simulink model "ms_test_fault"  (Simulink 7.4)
settings: Solver=ode23t  StartTime=0.0  StopTime=15  RelTol=1e-5
undefined symbols (not defined in the file or in its folder): D1, Delta, dfilt, DiscIntNeverNeededParam
libraries: powerlib x47, simulink x12, powerlib_extras x8, dsparch4 x3
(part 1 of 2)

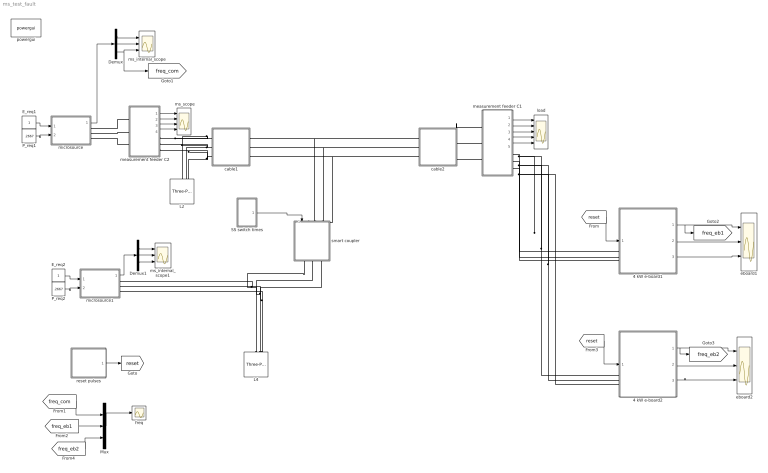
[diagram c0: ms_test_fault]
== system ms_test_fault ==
  " ms_scope" : Scope  NumInputPorts=4
  4 kW e-board1 : Subsystem  mask{tf=100, p=1}
      mask prompts: tf "fault_time"; p "load priority"
  4 kW e-board2 : Subsystem  mask{tf=100, p=2}
      mask prompts: tf "fault time"; p "priority level"
  Demux : Demux  Outputs=3
  Demux1 : Demux  Outputs=3
  E_req1 : Constant  OutDataType=fixdt(1, 16)  OutScaling=2^0
  E_req2 : Constant  OutDataType=fixdt(1, 16)  OutScaling=2^0
  L2 : powerlib/Elements/Three-Phase Series RLC Load  DialogController=POWERSYS.PowerSysDialog  PhysicalDomain=powersysdomain  SubClassName=unknown  LeftPortType=p1  RightPortType=p1  LConnTagsString=A|B|C  Configuration=Y (grounded)  NominalVoltage=208  NominalFrequency=60  ActivePower=4000  InductivePower=0  CapacitivePower=0  Measurements=None
  L4 : powerlib/Elements/Three-Phase Series RLC Load  DialogController=POWERSYS.PowerSysDialog  PhysicalDomain=powersysdomain  SubClassName=unknown  LeftPortType=p1  RightPortType=p1  LConnTagsString=A|B|C  Configuration=Y (grounded)  NominalVoltage=208  NominalFrequency=60  ActivePower=4000  InductivePower=0  CapacitivePower=0  Measurements=None
  Mux : Mux  Inputs=3
  P_req1 : Constant  Value=.2667  OutDataType=fixdt(1, 16)  OutScaling=2^0
  P_req2 : Constant  Value=.2667  OutDataType=fixdt(1, 16)  OutScaling=2^0
  SS switch times : Subsystem  mask{tdisconnect=3, dt=4}
      mask prompts: tdisconnect "disconnect time"; dt "disconnection interval"
  cable1 : Subsystem  mask{R=.002657, L=.000641, C=2020}
  cable2 : Subsystem  mask{R=0.0168, L=0.00407, C=336}
  eboard1 : Scope  NumInputPorts=3
  eboard2 : Scope  NumInputPorts=3
  freq : Scope
  load : Scope  NumInputPorts=5
  measurement feeder C1 : Subsystem
  measurement feeder C2 : Subsystem
  microsource : Subsystem  AncestorBlock=|
      | UWM_blocks/inverter-based
      | DG (simplified)
      | 208V - 15kVA
  microsource1 : Subsystem  AncestorBlock=|
      | UWM_blocks/inverter-based
      | DG (simplified)
      | 208V - 15kVA
  ms_internal_scope : Scope  NumInputPorts=3
  ms_internal_scope1 : Scope  NumInputPorts=3
  powergui : powerlib/powergui  Priority=1  SystemSampleTime=-1  SimulationMode=Discrete  SampleTime=50e-6  frequency=60  SPID=off  DisableSnubberDevices=off  DisableRonSwitches=off  DisableVfSwitches=off  SwTol=0  Interpol=off  frequencyindice=0  echomessages=off  HookPort=off  DisplayEquations=off  FunctionMessages=off  EnableUseOfTLC=off  x0status=blocks  RestoreLinks=warning  Frange=[0:2:500]  Ylog=off  Xlog=on  ShowGrid=off  save=off  variable=ZData  ZoomFFT=on  StartTime=0.0  cycles=1  DisplayStyle=1  fundamental=60  FreqAxis=off  MaxFrequency=1000  frequencyindicesteady=1  RmsSteady=1  display=off  Ts=0  methode=off
  reset pulses : Subsystem  mask{tpulse=[2 100]}
  smart coupler : Subsystem
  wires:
  measurement feeder C2/1(Vabc) -> " ms_scope"/1
  measurement feeder C2/2(Iabc) -> " ms_scope"/2
  measurement feeder C2/3(PQ) -> " ms_scope"/3
  measurement feeder C2/4(RMS (V-I)) -> " ms_scope"/4
  measurement feeder C1/5(w) -> load/5
  measurement feeder C1/4(RMS (V-I)) -> load/4
  measurement feeder C1/3(PQ) -> load/3
  measurement feeder C1/2(Iabc) -> load/2
  measurement feeder C1/1(Vabc) -> load/1
  P_req1/1 -> microsource/2(P_req)
  E_req1/1 -> microsource/1(E_req)
  Demux/2 -> ms_internal_scope/2
  Demux/1 -> ms_internal_scope/1
  Demux/3 -> ms_internal_scope/3, [freq_com]
  microsource/1(m) -> Demux/1
  Mux/1 -> freq/1
  P_req2/1 -> microsource1/2(P_req)
  E_req2/1 -> microsource1/1(E_req)
  microsource1/1(m) -> Demux1/1
  Demux1/1 -> ms_internal_scope1/1
  Demux1/2 -> ms_internal_scope1/2
  Demux1/3 -> ms_internal_scope1/3
  4 kW e-board1/1(w) -> eboard1/1, [freq_eb1]
  reset pulses/1(Out1) -> [reset]
  [reset] -> 4 kW e-board1/1(reset)
  [freq_com] -> Mux/1
  4 kW e-board1/2(Irms) -> eboard1/2
  4 kW e-board1/3(Vrms) -> eboard1/3
  [freq_eb1] -> Mux/2
  [reset] -> 4 kW e-board2/1(reset)
  4 kW e-board2/1(w) -> eboard2/1, [freq_eb2]
  4 kW e-board2/2(Irms) -> eboard2/2
  4 kW e-board2/3(Vrms) -> eboard2/3
  [freq_eb2] -> Mux/3
  SS switch times/1(Out1) -> smart coupler/1(switch)
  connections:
  cable1/RConn1 -- L2/LConn1 -- measurement feeder C2/RConn1
  cable1/RConn2 -- L2/LConn2 -- measurement feeder C2/RConn2
  cable1/RConn3 -- L2/LConn3 -- measurement feeder C2/RConn3
  microsource/RConn1 -- measurement feeder C2/LConn1
  microsource/RConn2 -- measurement feeder C2/LConn2
  microsource/RConn3 -- measurement feeder C2/LConn3
  cable2/LConn1 -- measurement feeder C1/LConn1
  cable2/LConn2 -- measurement feeder C1/LConn2
  cable2/LConn3 -- measurement feeder C1/LConn3
  measurement feeder C1/RConn1 -- 4 kW e-board1/LConn1 -- 4 kW e-board2/LConn1
  measurement feeder C1/RConn2 -- 4 kW e-board1/LConn2 -- 4 kW e-board2/LConn2
  measurement feeder C1/RConn3 -- 4 kW e-board1/LConn3 -- 4 kW e-board2/LConn3
  cable2/RConn2 -- cable1/LConn2 -- smart coupler/LConn2
  cable2/RConn3 -- cable1/LConn3 -- smart coupler/LConn3
  L4/LConn2 -- microsource1/RConn2 -- smart coupler/RConn2
  L4/LConn3 -- microsource1/RConn3 -- smart coupler/RConn3
  cable2/RConn1 -- cable1/LConn1 -- smart coupler/LConn1
  L4/LConn1 -- microsource1/RConn1 -- smart coupler/RConn1

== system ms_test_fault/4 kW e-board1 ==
  reset : Inport
  Current Measurement : powerlib/Measurements/Current Measurement  DialogController=POWERSYS.PowerSysDialog  SystemSampleTime=-1  PhasorSimulation=off  OutputType=Complex  PSBequivalent=0
  Ground : powerlib/Elements/Ground  DialogController=POWERSYS.PowerSysDialog  PhysicalDomain=powersysdomain  SubClassName=unknown  LeftPortType=p1  RightPortType=p1  LConnTagsString=a
  L1 : powerlib/Elements/Three-Phase Series RLC Load  DialogController=POWERSYS.PowerSysDialog  PhysicalDomain=powersysdomain  SubClassName=unknown  LeftPortType=p1  RightPortType=p1  LConnTagsString=A|B|C  Configuration=Y (grounded)  NominalVoltage=208  NominalFrequency=60  ActivePower=4000  InductivePower=0  CapacitivePower=0  Measurements=None
  Three-Phase Breaker2 : powerlib/Elements/Three-Phase Breaker  DialogController=POWERSYS.PowerSysDialog  SystemSampleTime=-1  InitialState=closed  SwitchA=on  SwitchB=on  SwitchC=on  SwitchTimes=[50]  External=on  BreakerResistance=0.001  SnubberResistance=1e6  SnubberCapacitance=inf  Measurements=None
  Three-Phase Fault : powerlib/Elements/Three-Phase Fault  DialogController=POWERSYS.PowerSysDialog  SystemSampleTime=-1  FaultA=on  FaultB=on  FaultC=on  FaultResistance=0.001  GroundFault=on  GroundResistance=0.001  External=off  SwitchStatus=[1 0]  SwitchTimes=[tf tf+3/60]  InitialStates=[0 0 1]  SnubberResistance=1e6  SnubberCapacitance=inf  Measurements=None
  Voltage  Measurement : powerlib/Measurements/Voltage Measurement  DialogController=POWERSYS.PowerSysDialog  SystemSampleTime=-1  PhasorSimulation=off  OutputType=Complex  PSBequivalent=0
  trip : Subsystem  mask{p=p}
      mask prompts: p "priority level"
  A : PMIOPort  Port=1  Side=Left
  B : PMIOPort  Port=2  Side=Left
  C : PMIOPort  Port=3  Side=Left
  w : Outport  OutDataType=fixdt(1, 16)  OutScaling=2^0
  Irms : Outport  Port=2  OutDataType=fixdt(1, 16)  OutScaling=2^0
  Vrms : Outport  Port=3  OutDataType=fixdt(1, 16)  OutScaling=2^0
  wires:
  trip/1(w) -> w/1
  Current Measurement/1 -> trip/3(I)
  Voltage  Measurement/1 -> trip/2(V)
  reset/1 -> trip/1(Reset)
  trip/2(trip) -> Three-Phase Breaker2/1
  trip/3(Irms) -> Irms/1
  trip/4(Vrms) -> Vrms/1
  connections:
  A/RConn1 -- Current Measurement/LConn1 -- Voltage  Measurement/LConn1
  Voltage  Measurement/LConn2 -- Ground/LConn1
  B/RConn1 -- Three-Phase Breaker2/LConn2
  Current Measurement/RConn1 -- Three-Phase Breaker2/LConn1
  C/RConn1 -- Three-Phase Breaker2/LConn3
  Three-Phase Breaker2/RConn1 -- Three-Phase Fault/LConn1 -- L1/LConn1
  Three-Phase Breaker2/RConn2 -- Three-Phase Fault/LConn2 -- L1/LConn2
  Three-Phase Breaker2/RConn3 -- Three-Phase Fault/LConn3 -- L1/LConn3

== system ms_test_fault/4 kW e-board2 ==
  reset : Inport
  Current Measurement : powerlib/Measurements/Current Measurement  DialogController=POWERSYS.PowerSysDialog  SystemSampleTime=-1  PhasorSimulation=off  OutputType=Complex  PSBequivalent=0
  Ground : powerlib/Elements/Ground  DialogController=POWERSYS.PowerSysDialog  PhysicalDomain=powersysdomain  SubClassName=unknown  LeftPortType=p1  RightPortType=p1  LConnTagsString=a
  L1 : powerlib/Elements/Three-Phase Series RLC Load  DialogController=POWERSYS.PowerSysDialog  PhysicalDomain=powersysdomain  SubClassName=unknown  LeftPortType=p1  RightPortType=p1  LConnTagsString=A|B|C  Configuration=Y (grounded)  NominalVoltage=208  NominalFrequency=60  ActivePower=4000  InductivePower=0  CapacitivePower=0  Measurements=None
  Three-Phase Breaker2 : powerlib/Elements/Three-Phase Breaker  DialogController=POWERSYS.PowerSysDialog  SystemSampleTime=-1  InitialState=closed  SwitchA=on  SwitchB=on  SwitchC=on  SwitchTimes=[50]  External=on  BreakerResistance=0.001  SnubberResistance=1e6  SnubberCapacitance=inf  Measurements=None
  Three-Phase Fault : powerlib/Elements/Three-Phase Fault  DialogController=POWERSYS.PowerSysDialog  SystemSampleTime=-1  FaultA=on  FaultB=on  FaultC=on  FaultResistance=0.001  GroundFault=on  GroundResistance=0.001  External=off  SwitchStatus=[1 0]  SwitchTimes=[tf tf+3/60]  InitialStates=[0 0 1]  SnubberResistance=1e6  SnubberCapacitance=inf  Measurements=None
  Voltage  Measurement : powerlib/Measurements/Voltage Measurement  DialogController=POWERSYS.PowerSysDialog  SystemSampleTime=-1  PhasorSimulation=off  OutputType=Complex  PSBequivalent=0
  trip : Subsystem  mask{p=p}
      mask prompts: p "priority level"
  A : PMIOPort  Port=1  Side=Left
  B : PMIOPort  Port=2  Side=Left
  C : PMIOPort  Port=3  Side=Left
  w : Outport  OutDataType=fixdt(1, 16)  OutScaling=2^0
  Irms : Outport  Port=2  OutDataType=fixdt(1, 16)  OutScaling=2^0
  Vrms : Outport  Port=3  OutDataType=fixdt(1, 16)  OutScaling=2^0
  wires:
  trip/1(w) -> w/1
  Current Measurement/1 -> trip/3(I)
  Voltage  Measurement/1 -> trip/2(V)
  reset/1 -> trip/1(Reset)
  trip/2(trip) -> Three-Phase Breaker2/1
  trip/3(Irms) -> Irms/1
  trip/4(Vrms) -> Vrms/1
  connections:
  A/RConn1 -- Current Measurement/LConn1 -- Voltage  Measurement/LConn1
  Voltage  Measurement/LConn2 -- Ground/LConn1
  B/RConn1 -- Three-Phase Breaker2/LConn2
  Current Measurement/RConn1 -- Three-Phase Breaker2/LConn1
  C/RConn1 -- Three-Phase Breaker2/LConn3
  Three-Phase Breaker2/RConn1 -- Three-Phase Fault/LConn1 -- L1/LConn1
  Three-Phase Breaker2/RConn2 -- Three-Phase Fault/LConn2 -- L1/LConn2
  Three-Phase Breaker2/RConn3 -- Three-Phase Fault/LConn3 -- L1/LConn3

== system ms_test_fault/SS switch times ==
  Sum : Sum  Inputs=|++  OutDataType=fixdt(1, 16)  OutScaling=2^0
  disconnect : Step  Time=tdisconnect  Before=1  After=0  SampleTime=0
  reconnect : Step  Time=tdisconnect+dt  SampleTime=0
  Out1 : Outport
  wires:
  reconnect/1 -> Sum/2
  disconnect/1 -> Sum/1
  Sum/1 -> Out1/1

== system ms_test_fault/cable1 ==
  Ground1 : powerlib/Elements/Ground  DialogController=POWERSYS.PowerSysDialog  PhysicalDomain=powersysdomain  SubClassName=unknown  LeftPortType=p1  RightPortType=p1  LConnTagsString=a
  Three-Phase Parallel RLC Branch : powerlib/Elements/Three-Phase Parallel RLC Branch  DialogController=POWERSYS.PowerSysDialog  PhysicalDomain=powersysdomain  SubClassName=unknown  LeftPortType=p1  RightPortType=p1  LConnTagsString=A|B|C  RConnTagsString=A|B|C  BranchType=C  Resistance=1  Inductance=1e-3  Capacitance=1/(C*2*pi*60)  Measurements=None
  Three-Phase Series RLC Branch3 : powerlib/Elements/Three-Phase Series RLC Branch  DialogController=POWERSYS.PowerSysDialog  PhysicalDomain=powersysdomain  SubClassName=unknown  LeftPortType=p1  RightPortType=p1  LConnTagsString=A|B|C  RConnTagsString=A|B|C  BranchType=RL  Resistance=R  Inductance=L/(2*pi*60)  Capacitance=1/(336*2*pi*60)  Measurements=None
  A* : PMIOPort  Tag=PMCPort  Port=1  Side=Right
  B* : PMIOPort  Tag=PMCPort  Port=2  Side=Right
  C* : PMIOPort  Tag=PMCPort  Port=3  Side=Right
  A : PMIOPort  Tag=PMCPort  Port=4  Side=Left
  B : PMIOPort  Tag=PMCPort  Port=5  Side=Left
  C : PMIOPort  Tag=PMCPort  Port=6  Side=Left
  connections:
  Three-Phase Parallel RLC Branch/RConn3 -- Ground1/LConn1 -- Three-Phase Parallel RLC Branch/RConn2 -- Three-Phase Parallel RLC Branch/RConn1
  Three-Phase Parallel RLC Branch/LConn1 -- A*/RConn1 -- Three-Phase Series RLC Branch3/LConn1
  Three-Phase Parallel RLC Branch/LConn2 -- B*/RConn1 -- Three-Phase Series RLC Branch3/LConn2
  Three-Phase Parallel RLC Branch/LConn3 -- C*/RConn1 -- Three-Phase Series RLC Branch3/LConn3
  A/RConn1 -- Three-Phase Series RLC Branch3/RConn1
  B/RConn1 -- Three-Phase Series RLC Branch3/RConn2
  C/RConn1 -- Three-Phase Series RLC Branch3/RConn3

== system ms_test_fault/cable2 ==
  Ground1 : powerlib/Elements/Ground  DialogController=POWERSYS.PowerSysDialog  PhysicalDomain=powersysdomain  SubClassName=unknown  LeftPortType=p1  RightPortType=p1  LConnTagsString=a
  Three-Phase Parallel RLC Branch : powerlib/Elements/Three-Phase Parallel RLC Branch  DialogController=POWERSYS.PowerSysDialog  PhysicalDomain=powersysdomain  SubClassName=unknown  LeftPortType=p1  RightPortType=p1  LConnTagsString=A|B|C  RConnTagsString=A|B|C  BranchType=C  Resistance=1  Inductance=1e-3  Capacitance=1/(C*2*pi*60)  Measurements=None
  Three-Phase Series RLC Branch3 : powerlib/Elements/Three-Phase Series RLC Branch  DialogController=POWERSYS.PowerSysDialog  PhysicalDomain=powersysdomain  SubClassName=unknown  LeftPortType=p1  RightPortType=p1  LConnTagsString=A|B|C  RConnTagsString=A|B|C  BranchType=RL  Resistance=R  Inductance=L/(2*pi*60)  Capacitance=1/(336*2*pi*60)  Measurements=None
  A* : PMIOPort  Tag=PMCPort  Port=1  Side=Right
  B* : PMIOPort  Tag=PMCPort  Port=2  Side=Right
  C* : PMIOPort  Tag=PMCPort  Port=3  Side=Right
  A : PMIOPort  Tag=PMCPort  Port=4  Side=Left
  B : PMIOPort  Tag=PMCPort  Port=5  Side=Left
  C : PMIOPort  Tag=PMCPort  Port=6  Side=Left
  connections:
  Three-Phase Parallel RLC Branch/RConn3 -- Ground1/LConn1 -- Three-Phase Parallel RLC Branch/RConn2 -- Three-Phase Parallel RLC Branch/RConn1
  Three-Phase Parallel RLC Branch/LConn1 -- A*/RConn1 -- Three-Phase Series RLC Branch3/LConn1
  Three-Phase Parallel RLC Branch/LConn2 -- B*/RConn1 -- Three-Phase Series RLC Branch3/LConn2
  Three-Phase Parallel RLC Branch/LConn3 -- C*/RConn1 -- Three-Phase Series RLC Branch3/LConn3
  A/RConn1 -- Three-Phase Series RLC Branch3/RConn1
  B/RConn1 -- Three-Phase Series RLC Branch3/RConn2
  C/RConn1 -- Three-Phase Series RLC Branch3/RConn3

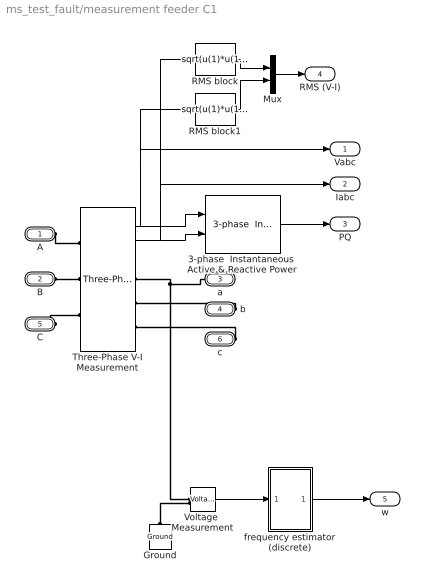
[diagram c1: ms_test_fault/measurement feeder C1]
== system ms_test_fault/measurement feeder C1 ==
  3-phase  Instantaneous  Active & Reactive Power : powerlib_extras/Measurements/3-phase  Instantaneous  Active & Reactive Power  DialogController=POWERSYS.PowerSysDialog  SystemSampleTime=-1
  Ground : powerlib/Elements/Ground  DialogController=POWERSYS.PowerSysDialog  PhysicalDomain=powersysdomain  SubClassName=unknown  LeftPortType=p1  RightPortType=p1  LConnTagsString=a
  Mux : Mux  Inputs=2
  RMS block : Fcn  Expr=sqrt(u(1)*u(1)+u(2)*u(2)+u(3)*u(3))/sqrt(3)
  RMS block1 : Fcn  Expr=sqrt(u(1)*u(1)+u(2)*u(2)+u(3)*u(3))/sqrt(3)
  Three-Phase V-I Measurement : powerlib/Measurements/Three-Phase V-I Measurement  DialogController=POWERSYS.PowerSysDialog  SystemSampleTime=-1  VoltageMeasurement=phase-to-ground  SetLabelV=off  LabelV=Vabc  Vpu=off  CurrentMeasurement=yes  SetLabelI=off  LabelI=Iabc  Ipu=off  Pbase=100e6  Vbase=500e3  OutputType=Complex  PhasorSimulation=off  PSBequivalent=0
  Voltage  Measurement : powerlib/Measurements/Voltage Measurement  DialogController=POWERSYS.PowerSysDialog  SystemSampleTime=-1  PhasorSimulation=off  OutputType=Complex  PSBequivalent=0
  frequency estimator (discrete) : Subsystem  mask{dt=0.010}
      mask prompts: dt "sample time"
  A : PMIOPort  Port=1  Side=Left
  B : PMIOPort  Port=2  Side=Left
  a : PMIOPort  Port=3  Side=Right
  b : PMIOPort  Port=4  Side=Right
  C : PMIOPort  Port=5  Side=Left
  c : PMIOPort  Port=6  Side=Right
  Vabc : Outport  OutDataType=fixdt(1, 16)  OutScaling=2^0
  Iabc : Outport  Port=2  OutDataType=fixdt(1, 16)  OutScaling=2^0
  PQ : Outport  Port=3  OutDataType=fixdt(1, 16)  OutScaling=2^0
  RMS (V-I) : Outport  Port=4  OutDataType=fixdt(1, 16)  OutScaling=2^0
  w : Outport  Port=5  OutDataType=fixdt(1, 16)  OutScaling=2^0
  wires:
  Three-Phase V-I Measurement/1 -> Vabc/1, RMS block1/1, 3-phase  Instantaneous  Active & Reactive Power/1
  Three-Phase V-I Measurement/2 -> Iabc/1, RMS block/1, 3-phase  Instantaneous  Active & Reactive Power/2
  Mux/1 -> RMS (V-I)/1
  RMS block/1 -> Mux/1
  RMS block1/1 -> Mux/2
  3-phase  Instantaneous  Active & Reactive Power/1 -> PQ/1
  Voltage  Measurement/1 -> frequency estimator (discrete)/1(In1)
  frequency estimator (discrete)/1(w) -> w/1
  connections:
  c/RConn1 -- Three-Phase V-I Measurement/RConn3
  C/RConn1 -- Three-Phase V-I Measurement/LConn3
  b/RConn1 -- Three-Phase V-I Measurement/RConn2
  Voltage  Measurement/LConn1 -- a/RConn1 -- Three-Phase V-I Measurement/RConn1
  B/RConn1 -- Three-Phase V-I Measurement/LConn2
  A/RConn1 -- Three-Phase V-I Measurement/LConn1
  Ground/LConn1 -- Voltage  Measurement/LConn2

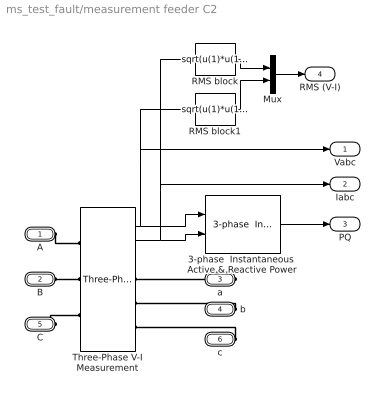
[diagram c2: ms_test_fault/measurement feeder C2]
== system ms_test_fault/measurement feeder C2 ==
  3-phase  Instantaneous  Active & Reactive Power : powerlib_extras/Measurements/3-phase  Instantaneous  Active & Reactive Power  DialogController=POWERSYS.PowerSysDialog  SystemSampleTime=-1
  Mux : Mux  Inputs=2
  RMS block : Fcn  Expr=sqrt(u(1)*u(1)+u(2)*u(2)+u(3)*u(3))/sqrt(3)
  RMS block1 : Fcn  Expr=sqrt(u(1)*u(1)+u(2)*u(2)+u(3)*u(3))/sqrt(3)
  Three-Phase V-I Measurement : powerlib/Measurements/Three-Phase V-I Measurement  DialogController=POWERSYS.PowerSysDialog  SystemSampleTime=-1  VoltageMeasurement=phase-to-ground  SetLabelV=off  LabelV=Vabc  Vpu=off  CurrentMeasurement=yes  SetLabelI=off  LabelI=Iabc  Ipu=off  Pbase=100e6  Vbase=500e3  OutputType=Complex  PhasorSimulation=off  PSBequivalent=0
  A : PMIOPort  Port=1  Side=Left
  B : PMIOPort  Port=2  Side=Left
  a : PMIOPort  Port=3  Side=Right
  b : PMIOPort  Port=4  Side=Right
  C : PMIOPort  Port=5  Side=Left
  c : PMIOPort  Port=6  Side=Right
  Vabc : Outport  OutDataType=fixdt(1, 16)  OutScaling=2^0
  Iabc : Outport  Port=2  OutDataType=fixdt(1, 16)  OutScaling=2^0
  PQ : Outport  Port=3  OutDataType=fixdt(1, 16)  OutScaling=2^0
  RMS (V-I) : Outport  Port=4  OutDataType=fixdt(1, 16)  OutScaling=2^0
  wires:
  Three-Phase V-I Measurement/1 -> Vabc/1, RMS block1/1, 3-phase  Instantaneous  Active & Reactive Power/1
  Three-Phase V-I Measurement/2 -> Iabc/1, RMS block/1, 3-phase  Instantaneous  Active & Reactive Power/2
  Mux/1 -> RMS (V-I)/1
  RMS block/1 -> Mux/1
  RMS block1/1 -> Mux/2
  3-phase  Instantaneous  Active & Reactive Power/1 -> PQ/1
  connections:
  c/RConn1 -- Three-Phase V-I Measurement/RConn3
  C/RConn1 -- Three-Phase V-I Measurement/LConn3
  b/RConn1 -- Three-Phase V-I Measurement/RConn2
  a/RConn1 -- Three-Phase V-I Measurement/RConn1
  B/RConn1 -- Three-Phase V-I Measurement/LConn2
  A/RConn1 -- Three-Phase V-I Measurement/LConn1

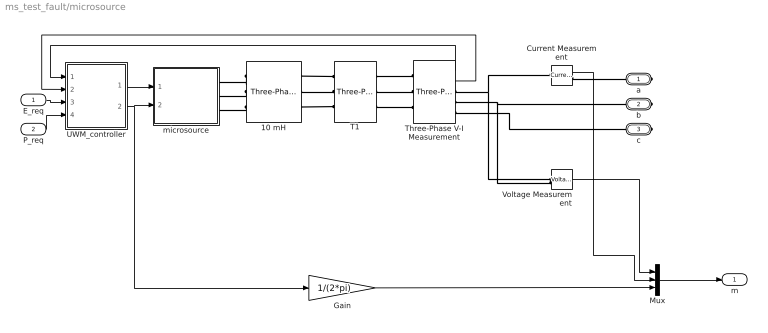
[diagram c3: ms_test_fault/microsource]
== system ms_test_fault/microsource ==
  E_req : Inport
  P_req : Inport  Port=2
  10 mH : powerlib/Elements/Three-Phase Series RLC Branch  DialogController=POWERSYS.PowerSysDialog  PhysicalDomain=powersysdomain  SubClassName=unknown  LeftPortType=p1  RightPortType=p1  LConnTagsString=A|B|C  RConnTagsString=A|B|C  BranchType=L  Resistance=.0028  Inductance=5e-3  Capacitance=1e-6  Measurements=None
  Current Measurement : powerlib/Measurements/Current Measurement  DialogController=POWERSYS.PowerSysDialog  SystemSampleTime=-1  PhasorSimulation=off  OutputType=Complex  PSBequivalent=0
  Gain : Gain  Gain=1/(2*pi)  ParameterDataType=fixdt(1, 16)  ParameterScaling=2^0  OutDataType=fixdt(1, 16)  OutScaling=2^0
  Mux : Mux  Inputs=3
  T1 : powerlib/Elements/Three-Phase Transformer (Two Windings)  DialogController=POWERSYS.PowerSysDialog  SystemSampleTime=-1  Winding1Connection=Delta (D1)  UNITS=SI  NominalPower=[ 45e3 , 60 ]  Winding1=[208 0.02688 0.1075/(2*pi*60)]  Winding2Connection=Yg  Winding2=[208 0.005047 .0201/(2*pi*60)]  SetSaturation=off  Rm=100.e6  Lm=7650.8  Saturation=[0 0;1359.8 0.93633;5.6659e+05 1.186]  Hysteresis=off  DataFile='hysteresis'  SetInitialFlux=off  InitialFluxes=[0.62422 -0.62422 0.54618]  Measurements=None  MoreParameters=off  BreakLoop=off  DataType=on  TransfoNumber=1
  Three-Phase V-I Measurement : powerlib/Measurements/Three-Phase V-I Measurement  DialogController=POWERSYS.PowerSysDialog  SystemSampleTime=-1  VoltageMeasurement=phase-to-ground  SetLabelV=off  LabelV=Vabc  Vpu=off  CurrentMeasurement=yes  SetLabelI=off  LabelI=Iabc  Ipu=off  Pbase=100e6  Vbase=500e3  OutputType=Complex  PhasorSimulation=off  PSBequivalent=0
  UWM_controller : Subsystem  mask{Vbase=208, Sbase=15000}
  Voltage Measurement : powerlib/Measurements/Voltage Measurement  DialogController=POWERSYS.PowerSysDialog  SystemSampleTime=-1  PhasorSimulation=off  OutputType=Complex  PSBequivalent=0
  microsource : Subsystem
  a : PMIOPort  Port=1  Side=Right
  b : PMIOPort  Port=2  Side=Right
  c : PMIOPort  Port=3  Side=Right
  m : Outport  OutDataType=fixdt(1, 16)  OutScaling=2^0
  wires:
  E_req/1 -> UWM_controller/3(E_req)
  P_req/1 -> UWM_controller/4(P_req)
  Three-Phase V-I Measurement/1 -> UWM_controller/1(v_meas)
  Three-Phase V-I Measurement/2 -> UWM_controller/2(i_meas)
  UWM_controller/1(Vpk) -> microsource/1(Vpk)
  UWM_controller/2(w) -> microsource/2(w), Gain/1
  Mux/1 -> m/1
  Voltage Measurement/1 -> Mux/1
  Current Measurement/1 -> Mux/2
  Gain/1 -> Mux/3
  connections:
  Three-Phase V-I Measurement/RConn2 -- b/RConn1 -- Voltage Measurement/LConn2
  Three-Phase V-I Measurement/RConn3 -- c/RConn1
  Current Measurement/RConn1 -- a/RConn1
  Three-Phase V-I Measurement/RConn1 -- Current Measurement/LConn1 -- Voltage Measurement/LConn1
  10 mH/LConn2 -- microsource/RConn2
  10 mH/LConn1 -- microsource/RConn1
  10 mH/LConn3 -- microsource/RConn3
  T1/LConn1 -- 10 mH/RConn1
  T1/LConn2 -- 10 mH/RConn2
  T1/LConn3 -- 10 mH/RConn3
  T1/RConn1 -- Three-Phase V-I Measurement/LConn1
  T1/RConn2 -- Three-Phase V-I Measurement/LConn2
  T1/RConn3 -- Three-Phase V-I Measurement/LConn3

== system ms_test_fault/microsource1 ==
  E_req : Inport
  P_req : Inport  Port=2
  10 mH : powerlib/Elements/Three-Phase Series RLC Branch  DialogController=POWERSYS.PowerSysDialog  PhysicalDomain=powersysdomain  SubClassName=unknown  LeftPortType=p1  RightPortType=p1  LConnTagsString=A|B|C  RConnTagsString=A|B|C  BranchType=L  Resistance=.0028  Inductance=5e-3  Capacitance=1e-6  Measurements=None
  Current Measurement : powerlib/Measurements/Current Measurement  DialogController=POWERSYS.PowerSysDialog  SystemSampleTime=-1  PhasorSimulation=off  OutputType=Complex  PSBequivalent=0
  Gain : Gain  Gain=1/(2*pi)  ParameterDataType=fixdt(1, 16)  ParameterScaling=2^0  OutDataType=fixdt(1, 16)  OutScaling=2^0
  Mux : Mux  Inputs=3
  T1 : powerlib/Elements/Three-Phase Transformer (Two Windings)  DialogController=POWERSYS.PowerSysDialog  SystemSampleTime=-1  Winding1Connection=Delta (D1)  UNITS=SI  NominalPower=[ 45e3 , 60 ]  Winding1=[208 0.02688 0.1075/(2*pi*60)]  Winding2Connection=Yg  Winding2=[208 0.005047 .0201/(2*pi*60)]  SetSaturation=off  Rm=100.e6  Lm=7650.8  Saturation=[0 0;1359.8 0.93633;5.6659e+05 1.186]  Hysteresis=off  DataFile='hysteresis'  SetInitialFlux=off  InitialFluxes=[0.62422 -0.62422 0.54618]  Measurements=None  MoreParameters=off  BreakLoop=off  DataType=on  TransfoNumber=1
  Three-Phase V-I Measurement : powerlib/Measurements/Three-Phase V-I Measurement  DialogController=POWERSYS.PowerSysDialog  SystemSampleTime=-1  VoltageMeasurement=phase-to-ground  SetLabelV=off  LabelV=Vabc  Vpu=off  CurrentMeasurement=yes  SetLabelI=off  LabelI=Iabc  Ipu=off  Pbase=100e6  Vbase=500e3  OutputType=Complex  PhasorSimulation=off  PSBequivalent=0
  UWM_controller : Subsystem  mask{Vbase=208, Sbase=15000}
  Voltage Measurement : powerlib/Measurements/Voltage Measurement  DialogController=POWERSYS.PowerSysDialog  SystemSampleTime=-1  PhasorSimulation=off  OutputType=Complex  PSBequivalent=0
  microsource : Subsystem
  a : PMIOPort  Port=1  Side=Right
  b : PMIOPort  Port=2  Side=Right
  c : PMIOPort  Port=3  Side=Right
  m : Outport  OutDataType=fixdt(1, 16)  OutScaling=2^0
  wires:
  E_req/1 -> UWM_controller/3(E_req)
  P_req/1 -> UWM_controller/4(P_req)
  Three-Phase V-I Measurement/1 -> UWM_controller/1(v_meas)
  Three-Phase V-I Measurement/2 -> UWM_controller/2(i_meas)
  UWM_controller/1(Vpk) -> microsource/1(Vpk)
  UWM_controller/2(w) -> microsource/2(w), Gain/1
  Mux/1 -> m/1
  Voltage Measurement/1 -> Mux/1
  Current Measurement/1 -> Mux/2
  Gain/1 -> Mux/3
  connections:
  Three-Phase V-I Measurement/RConn2 -- b/RConn1 -- Voltage Measurement/LConn2
  Three-Phase V-I Measurement/RConn3 -- c/RConn1
  Current Measurement/RConn1 -- a/RConn1
  Three-Phase V-I Measurement/RConn1 -- Current Measurement/LConn1 -- Voltage Measurement/LConn1
  10 mH/LConn2 -- microsource/RConn2
  10 mH/LConn1 -- microsource/RConn1
  10 mH/LConn3 -- microsource/RConn3
  T1/LConn1 -- 10 mH/RConn1
  T1/LConn2 -- 10 mH/RConn2
  T1/LConn3 -- 10 mH/RConn3
  T1/RConn1 -- Three-Phase V-I Measurement/LConn1
  T1/RConn2 -- Three-Phase V-I Measurement/LConn2
  T1/RConn3 -- Three-Phase V-I Measurement/LConn3

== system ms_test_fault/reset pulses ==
  Sum : Sum  Inputs=|++  OutDataType=fixdt(1, 16)  OutScaling=2^0
  pulse : Subsystem  mask{tstart=tpulse(1), dt=.1}
  pulse1 : Subsystem  mask{tstart=tpulse(2), dt=.1}
  Out1 : Outport
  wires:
  pulse/1(Out1) -> Sum/1
  pulse1/1(Out1) -> Sum/2
  Sum/1 -> Out1/1

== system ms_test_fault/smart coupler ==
  switch : Inport  OutDataType=fixdt(1, 16)  OutScaling=2^0
  Abs : Abs  OutDataType=fixdt(1, 16)  OutScaling=2^0
  Level-2 M-file S-Function : M-S-Function  FunctionName=smart_coupler
  Mux : Mux  Inputs=2
  SS2 : powerlib/Elements/Three-Phase Breaker  DialogController=POWERSYS.PowerSysDialog  SystemSampleTime=-1  InitialState=closed  SwitchA=on  SwitchB=on  SwitchC=on  SwitchTimes=[5 6]  External=on  BreakerResistance=.001  SnubberResistance=1e6  SnubberCapacitance=inf  Measurements=None
  Scope : Scope  NumInputPorts=3
  Transfer Fcn : TransferFcn  Numerator=[10]  Denominator=[1 10]
  Voltage Measurement : powerlib/Measurements/Voltage Measurement  DialogController=POWERSYS.PowerSysDialog  SystemSampleTime=-1  PhasorSimulation=off  OutputType=Complex  PSBequivalent=0
  A : PMIOPort  Port=1  Side=Left
  B : PMIOPort  Port=2  Side=Left
  C : PMIOPort  Port=3  Side=Left
  a : PMIOPort  Port=4  Side=Right
  b : PMIOPort  Port=5  Side=Right
  c : PMIOPort  Port=6  Side=Right
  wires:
  switch/1 -> Level-2 M-file S-Function/2, Scope/2
  Level-2 M-file S-Function/1 -> Scope/1, SS2/1
  Voltage Measurement/1 -> Abs/1
  Abs/1 -> Transfer Fcn/1
  Transfer Fcn/1 -> Level-2 M-file S-Function/1, Mux/1
  Mux/1 -> Scope/3
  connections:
  A/RConn1 -- SS2/LConn1 -- Voltage Measurement/LConn1
  Voltage Measurement/LConn2 -- a/RConn1 -- SS2/RConn1
  B/RConn1 -- SS2/LConn2
  C/RConn1 -- SS2/LConn3
  b/RConn1 -- SS2/RConn2
  c/RConn1 -- SS2/RConn3

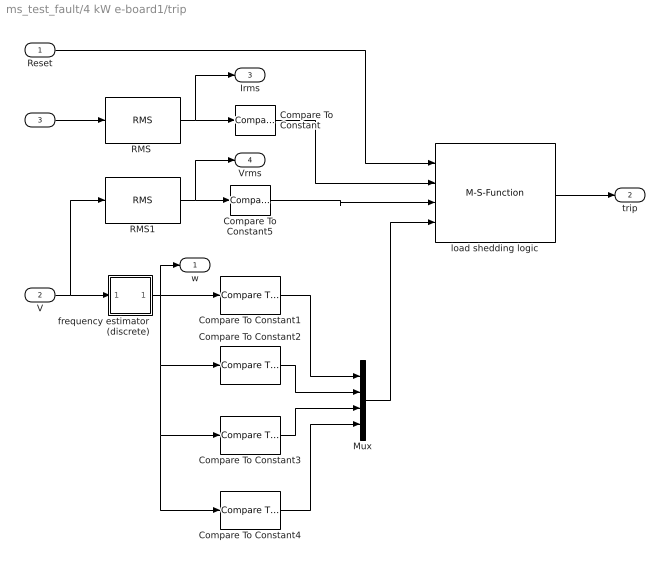
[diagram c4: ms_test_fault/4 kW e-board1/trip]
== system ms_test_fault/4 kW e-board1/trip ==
  Reset : Inport
  V : Inport  Port=2
  I : Inport  Port=3
  Compare To Constant : simulink/Logic and Bit Operations/Compare To Constant  SystemSampleTime=-1  relop=>=  const=100  LogicOutDataTypeMode=boolean
  Compare To Constant1 : simulink/Logic and Bit Operations/Compare To Constant  SystemSampleTime=-1  relop=<=  const=59.8  LogicOutDataTypeMode=boolean
  Compare To Constant2 : simulink/Logic and Bit Operations/Compare To Constant  SystemSampleTime=-1  relop=<=  const=59.5  LogicOutDataTypeMode=boolean
  Compare To Constant3 : simulink/Logic and Bit Operations/Compare To Constant  SystemSampleTime=-1  relop=>=  const=59.9  LogicOutDataTypeMode=boolean
  Compare To Constant4 : simulink/Logic and Bit Operations/Compare To Constant  SystemSampleTime=-1  relop=<=  const=58.6  LogicOutDataTypeMode=boolean
  Compare To Constant5 : simulink/Logic and Bit Operations/Compare To Constant  SystemSampleTime=-1  relop=<=  const=100  LogicOutDataTypeMode=boolean
  Mux : Mux
  "RMS " : powerlib_extras/Measurements/RMS  DialogController=POWERSYS.PowerSysDialog  SystemSampleTime=-1  f1=60
  RMS1 : powerlib_extras/Measurements/RMS  DialogController=POWERSYS.PowerSysDialog  SystemSampleTime=-1  f1=60
  frequency estimator (discrete) : Subsystem  mask{dt=0.010}
      mask prompts: dt "sample time"
  load shedding logic : M-S-Function  FunctionName=load_shedding_logic  Parameters=p
  w : Outport  OutDataType=fixdt(1, 16)  OutScaling=2^0
  trip : Outport  Port=2
  Irms : Outport  Port=3  OutDataType=fixdt(1, 16)  OutScaling=2^0
  Vrms : Outport  Port=4  OutDataType=fixdt(1, 16)  OutScaling=2^0
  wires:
  "RMS "/1 -> Compare To Constant/1, Irms/1
  I/1 -> "RMS "/1
  Reset/1 -> load shedding logic/1
  Compare To Constant/1 -> load shedding logic/2
  load shedding logic/1 -> trip/1
  V/1 -> frequency estimator (discrete)/1(v), RMS1/1
  frequency estimator (discrete)/1(w) -> Compare To Constant1/1, w/1, Compare To Constant2/1, Compare To Constant3/1, Compare To Constant4/1
  Compare To Constant1/1 -> Mux/1
  Compare To Constant2/1 -> Mux/2
  Compare To Constant3/1 -> Mux/3
  Compare To Constant4/1 -> Mux/4
  RMS1/1 -> Compare To Constant5/1, Vrms/1
  Compare To Constant5/1 -> load shedding logic/3
  Mux/1 -> load shedding logic/4

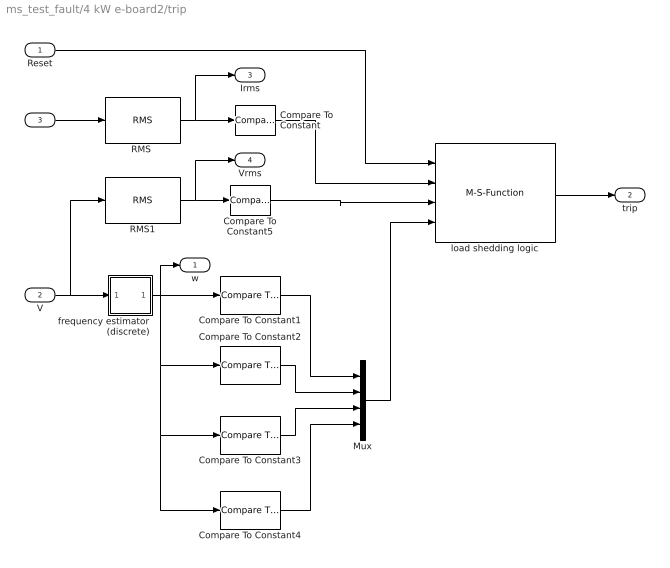
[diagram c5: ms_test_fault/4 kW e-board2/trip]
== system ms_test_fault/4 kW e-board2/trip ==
  Reset : Inport
  V : Inport  Port=2
  I : Inport  Port=3
  Compare To Constant : simulink/Logic and Bit Operations/Compare To Constant  SystemSampleTime=-1  relop=>=  const=100  LogicOutDataTypeMode=boolean
  Compare To Constant1 : simulink/Logic and Bit Operations/Compare To Constant  SystemSampleTime=-1  relop=<=  const=59.8  LogicOutDataTypeMode=boolean
  Compare To Constant2 : simulink/Logic and Bit Operations/Compare To Constant  SystemSampleTime=-1  relop=<=  const=59.5  LogicOutDataTypeMode=boolean
  Compare To Constant3 : simulink/Logic and Bit Operations/Compare To Constant  SystemSampleTime=-1  relop=>=  const=59.9  LogicOutDataTypeMode=boolean
  Compare To Constant4 : simulink/Logic and Bit Operations/Compare To Constant  SystemSampleTime=-1  relop=<=  const=58.6  LogicOutDataTypeMode=boolean
  Compare To Constant5 : simulink/Logic and Bit Operations/Compare To Constant  SystemSampleTime=-1  relop=<=  const=100  LogicOutDataTypeMode=boolean
  Mux : Mux
  "RMS " : powerlib_extras/Measurements/RMS  DialogController=POWERSYS.PowerSysDialog  SystemSampleTime=-1  f1=60
  RMS1 : powerlib_extras/Measurements/RMS  DialogController=POWERSYS.PowerSysDialog  SystemSampleTime=-1  f1=60
  frequency estimator (discrete) : Subsystem  mask{dt=0.010}
      mask prompts: dt "sample time"
  load shedding logic : M-S-Function  FunctionName=load_shedding_logic  Parameters=p
  w : Outport  OutDataType=fixdt(1, 16)  OutScaling=2^0
  trip : Outport  Port=2
  Irms : Outport  Port=3  OutDataType=fixdt(1, 16)  OutScaling=2^0
  Vrms : Outport  Port=4  OutDataType=fixdt(1, 16)  OutScaling=2^0
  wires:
  "RMS "/1 -> Compare To Constant/1, Irms/1
  I/1 -> "RMS "/1
  Reset/1 -> load shedding logic/1
  Compare To Constant/1 -> load shedding logic/2
  load shedding logic/1 -> trip/1
  V/1 -> frequency estimator (discrete)/1(v), RMS1/1
  frequency estimator (discrete)/1(w) -> Compare To Constant1/1, w/1, Compare To Constant2/1, Compare To Constant3/1, Compare To Constant4/1
  Compare To Constant1/1 -> Mux/1
  Compare To Constant2/1 -> Mux/2
  Compare To Constant3/1 -> Mux/3
  Compare To Constant4/1 -> Mux/4
  RMS1/1 -> Compare To Constant5/1, Vrms/1
  Compare To Constant5/1 -> load shedding logic/3
  Mux/1 -> load shedding logic/4

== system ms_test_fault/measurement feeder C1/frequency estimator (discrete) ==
  In1 : Inport
  Constant : Constant  Value=60  OutDataType=fixdt(1, 16)  OutScaling=2^0
  Fcn : Fcn  Expr=sin(2*pi*u[1])
  Filter1 : dsparch4/Biquad Filter  Tag=BlockMethodSubSystem  DialogController=dspdialog.BiquadFilter  DialogControllerArgs=DataTag2  IIRFiltStruct=Direct form II  CoeffSource=Specify via dialog  BiQuadCoeffs=[1 -1.36 1 1 -1.78 0.87;1 1 0 1 -0.85 0]  a0Flag=Warning  IC=0  ICnum=0  ICden=0  denAccumFracLength=30  denProdOutputFracLength=30  secondMemoryFracLength=15  roundingMode=Floor  overflowMode=off  ScaleValues=[0.05;0.23;1]  optimizeScaleValues=on  ScaleValueMode=Specify via input port (g)  scaleValueFracLength=14  FilterSource=Specify via dialog  dfiltObjectName=dfilt.df2tsos([1 0.3 0.4],[1 0.1 0.2])
  Gain : Gain  Gain=1/150  ParameterDataType=fixdt(1, 16)  ParameterScaling=2^0  OutDataType=fixdt(1, 16)  OutScaling=2^0  SampleTime=dt
  Product : Product  OutDataType=fixdt(1, 16)  OutScaling=2^0
  Scope : Scope
  Sum : Sum  Inputs=|++  OutDataType=fixdt(1, 16)  OutScaling=2^0
  modulo discrete integrator : Subsystem  mask{dt=dt}
      mask prompts: dt "sample time"
  w : Outport  OutDataType=fixdt(1, 16)  OutScaling=2^0
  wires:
  Fcn/1 -> Product/2
  Gain/1 -> Product/1
  Constant/1 -> Sum/2
  modulo discrete integrator/1(Out1) -> Fcn/1
  Sum/1 -> modulo discrete integrator/1(In1), w/1
  In1/1 -> Gain/1
  Product/1 -> Filter1/1
  Filter1/1 -> Scope/1, Sum/1

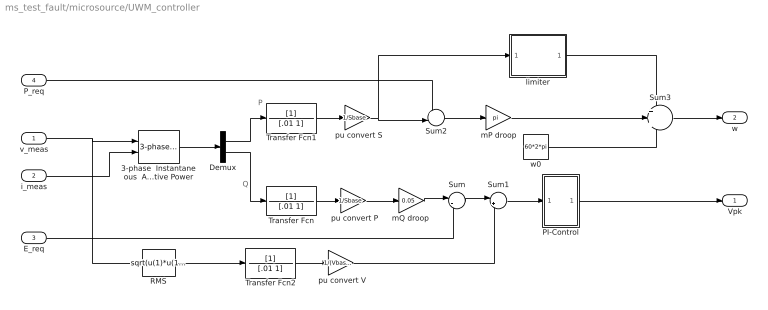
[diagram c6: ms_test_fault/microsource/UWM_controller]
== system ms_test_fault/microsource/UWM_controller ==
  note: P
  note: Q
  v_meas : Inport
  i_meas : Inport  Port=2
  E_req : Inport  Port=3
  P_req : Inport  Port=4
  " pu convert P" : Gain  Gain=1/Sbase  ParameterDataType=sfix(16)  ParameterScaling=2^0  OutDataType=sfix(16)  OutScaling=2^0
  " pu convert S" : Gain  Gain=1/Sbase  ParameterDataType=sfix(16)  ParameterScaling=2^0  OutDataType=sfix(16)  OutScaling=2^0
  " pu convert V" : Gain  Gain=1/(Vbase/sqrt(3))  ParameterDataType=sfix(16)  ParameterScaling=2^0  OutDataType=sfix(16)  OutScaling=2^0
  3-phase  Instantaneous  Active & Reactive Power : powerlib_extras/Measurements/3-phase  Instantaneous  Active & Reactive Power  DialogController=POWERSYS.PowerSysDialog  SystemSampleTime=-1
  Demux : Demux  Outputs=2
  PI-Control : Subsystem
  RMS : Fcn  Expr=sqrt(u(1)*u(1)+u(2)*u(2)+u(3)*u(3))/sqrt(3)
  Sum : Sum  Inputs=|-+  OutDataType=sfix(16)  OutScaling=2^0
  Sum1 : Sum  Inputs=|+-  OutDataType=sfix(16)  OutScaling=2^0
  Sum2 : Sum  Inputs=+-|  OutDataType=sfix(16)  OutScaling=2^0
  Sum3 : Sum  Inputs=+++  OutDataType=sfix(16)  OutScaling=2^0
  Transfer Fcn : TransferFcn  Denominator=[.01 1]
  Transfer Fcn1 : TransferFcn  Denominator=[.01 1]
  Transfer Fcn2 : TransferFcn  Denominator=[.01 1]
  limiter : Subsystem
  mP droop : Gain  Gain=pi  ParameterDataType=sfix(16)  ParameterScaling=2^0  OutDataType=sfix(16)  OutScaling=2^0
  "mQ droop " : Gain  Gain=0.05  ParameterDataType=sfix(16)  ParameterScaling=2^0  OutDataType=sfix(16)  OutScaling=2^0
  w0 : Constant  Value=60*2*pi  OutDataType=fixdt(1, 16)  OutScaling=2^0
  Vpk : Outport
  w : Outport  Port=2
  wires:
  Transfer Fcn2/1 -> " pu convert V"/1
  Transfer Fcn/1 -> " pu convert P"/1
  " pu convert P"/1 -> "mQ droop "/1
  Transfer Fcn1/1 -> " pu convert S"/1
  " pu convert S"/1 -> limiter/1(In1), Sum2/2
  i_meas/1 -> 3-phase  Instantaneous  Active & Reactive Power/2
  P_req/1 -> Sum2/1
  mP droop/1 -> Sum3/2
  limiter/1(Out1) -> Sum3/1
  w0/1 -> Sum3/3
  Sum2/1 -> mP droop/1
  Sum1/1 -> PI-Control/1(In1)
  Sum/1 -> Sum1/1
  "mQ droop "/1 -> Sum/1
  RMS/1 -> Transfer Fcn2/1
  Demux/2 -> Transfer Fcn/1
  Demux/1 -> Transfer Fcn1/1
  3-phase  Instantaneous  Active & Reactive Power/1 -> Demux/1
  v_meas/1 -> RMS/1, 3-phase  Instantaneous  Active & Reactive Power/1
  PI-Control/1(Out1) -> Vpk/1
  Sum3/1 -> w/1
  E_req/1 -> Sum/2
  " pu convert V"/1 -> Sum1/2

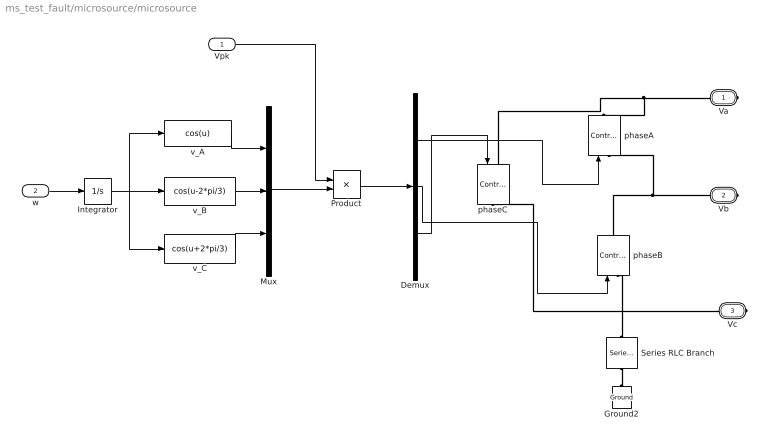
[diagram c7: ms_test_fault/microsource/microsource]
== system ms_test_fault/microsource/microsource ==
  Vpk : Inport  OutDataType=fixdt(1, 16)  OutScaling=2^0
  w : Inport  Port=2  OutDataType=fixdt(1, 16)  OutScaling=2^0
  Demux : Demux  Outputs=3
  Ground2 : powerlib/Elements/Ground  DialogController=POWERSYS.PowerSysDialog  PhysicalDomain=powersysdomain  SubClassName=unknown  LeftPortType=p1  RightPortType=p1  LConnTagsString=a
  Integrator : Integrator
  Mux : Mux  Inputs=3
  Product : Product  OutDataType=sfix(16)  OutScaling=2^0
  Series RLC Branch : powerlib/Elements/Series RLC Branch  DialogController=POWERSYS.PowerSysDialog  PhysicalDomain=powersysdomain  SubClassName=unknown  LeftPortType=p1  RightPortType=p1  LConnTagsString=__new0  RConnTagsString=__new0  BranchType=C  Resistance=1  Inductance=1e-3  SetiL0=off  InitialCurrent=0  Capacitance=1e-8  Setx0=off  InitialVoltage=0  Measurements=None
  phaseA : powerlib/Electrical Sources/Controlled Voltage Source  DialogController=POWERSYS.PowerSysDialog  SystemSampleTime=-1  Initialize=on  Source_Type=AC  Amplitude=0  Phase=0  Frequency=0  Measurements=None
  phaseB : powerlib/Electrical Sources/Controlled Voltage Source  DialogController=POWERSYS.PowerSysDialog  SystemSampleTime=-1  Initialize=on  Source_Type=AC  Amplitude=0  Phase=0  Frequency=0  Measurements=None
  phaseC : powerlib/Electrical Sources/Controlled Voltage Source  DialogController=POWERSYS.PowerSysDialog  SystemSampleTime=-1  Initialize=on  Source_Type=AC  Amplitude=0  Phase=0  Frequency=0  Measurements=None
  v_A : Fcn  Expr=cos(u)
  v_B : Fcn  Expr=cos(u-2*pi/3)
  v_C : Fcn  Expr=cos(u+2*pi/3)
  Va : PMIOPort  Tag=PMCPort  Port=1  Side=Right
  Vb : PMIOPort  Tag=PMCPort  Port=2  Side=Right
  Vc : PMIOPort  Tag=PMCPort  Port=3  Side=Right
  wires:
  Product/1 -> Demux/1
  Vpk/1 -> Product/1
  Mux/1 -> Product/2
  w/1 -> Integrator/1
  Integrator/1 -> v_A/1, v_B/1, v_C/1
  v_A/1 -> Mux/1
  v_B/1 -> Mux/2
  v_C/1 -> Mux/3
  Demux/1 -> phaseA/1
  Demux/2 -> phaseB/1
  Demux/3 -> phaseC/1
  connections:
  Vb/RConn1 -- phaseB/RConn1 -- phaseA/LConn1
  Va/RConn1 -- phaseC/LConn1 -- phaseA/RConn1
  Vc/RConn1 -- phaseC/RConn1
  Series RLC Branch/RConn1 -- Ground2/LConn1
  Series RLC Branch/LConn1 -- phaseB/LConn1

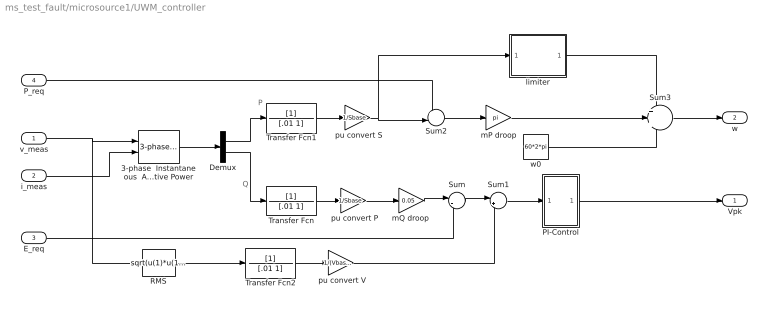
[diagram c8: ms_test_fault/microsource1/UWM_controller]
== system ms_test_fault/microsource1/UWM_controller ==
  note: P
  note: Q
  v_meas : Inport
  i_meas : Inport  Port=2
  E_req : Inport  Port=3
  P_req : Inport  Port=4
  " pu convert P" : Gain  Gain=1/Sbase  ParameterDataType=sfix(16)  ParameterScaling=2^0  OutDataType=sfix(16)  OutScaling=2^0
  " pu convert S" : Gain  Gain=1/Sbase  ParameterDataType=sfix(16)  ParameterScaling=2^0  OutDataType=sfix(16)  OutScaling=2^0
  " pu convert V" : Gain  Gain=1/(Vbase/sqrt(3))  ParameterDataType=sfix(16)  ParameterScaling=2^0  OutDataType=sfix(16)  OutScaling=2^0
  3-phase  Instantaneous  Active & Reactive Power : powerlib_extras/Measurements/3-phase  Instantaneous  Active & Reactive Power  DialogController=POWERSYS.PowerSysDialog  SystemSampleTime=-1
  Demux : Demux  Outputs=2
  PI-Control : Subsystem
  RMS : Fcn  Expr=sqrt(u(1)*u(1)+u(2)*u(2)+u(3)*u(3))/sqrt(3)
  Sum : Sum  Inputs=|-+  OutDataType=sfix(16)  OutScaling=2^0
  Sum1 : Sum  Inputs=|+-  OutDataType=sfix(16)  OutScaling=2^0
  Sum2 : Sum  Inputs=+-|  OutDataType=sfix(16)  OutScaling=2^0
  Sum3 : Sum  Inputs=+++  OutDataType=sfix(16)  OutScaling=2^0
  Transfer Fcn : TransferFcn  Denominator=[.01 1]
  Transfer Fcn1 : TransferFcn  Denominator=[.01 1]
  Transfer Fcn2 : TransferFcn  Denominator=[.01 1]
  limiter : Subsystem
  mP droop : Gain  Gain=pi  ParameterDataType=sfix(16)  ParameterScaling=2^0  OutDataType=sfix(16)  OutScaling=2^0
  "mQ droop " : Gain  Gain=0.05  ParameterDataType=sfix(16)  ParameterScaling=2^0  OutDataType=sfix(16)  OutScaling=2^0
  w0 : Constant  Value=60*2*pi  OutDataType=fixdt(1, 16)  OutScaling=2^0
  Vpk : Outport
  w : Outport  Port=2
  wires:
  Transfer Fcn2/1 -> " pu convert V"/1
  Transfer Fcn/1 -> " pu convert P"/1
  " pu convert P"/1 -> "mQ droop "/1
  Transfer Fcn1/1 -> " pu convert S"/1
  " pu convert S"/1 -> limiter/1(In1), Sum2/2
  i_meas/1 -> 3-phase  Instantaneous  Active & Reactive Power/2
  P_req/1 -> Sum2/1
  mP droop/1 -> Sum3/2
  limiter/1(Out1) -> Sum3/1
  w0/1 -> Sum3/3
  Sum2/1 -> mP droop/1
  Sum1/1 -> PI-Control/1(In1)
  Sum/1 -> Sum1/1
  "mQ droop "/1 -> Sum/1
  RMS/1 -> Transfer Fcn2/1
  Demux/2 -> Transfer Fcn/1
  Demux/1 -> Transfer Fcn1/1
  3-phase  Instantaneous  Active & Reactive Power/1 -> Demux/1
  v_meas/1 -> RMS/1, 3-phase  Instantaneous  Active & Reactive Power/1
  PI-Control/1(Out1) -> Vpk/1
  Sum3/1 -> w/1
  E_req/1 -> Sum/2
  " pu convert V"/1 -> Sum1/2

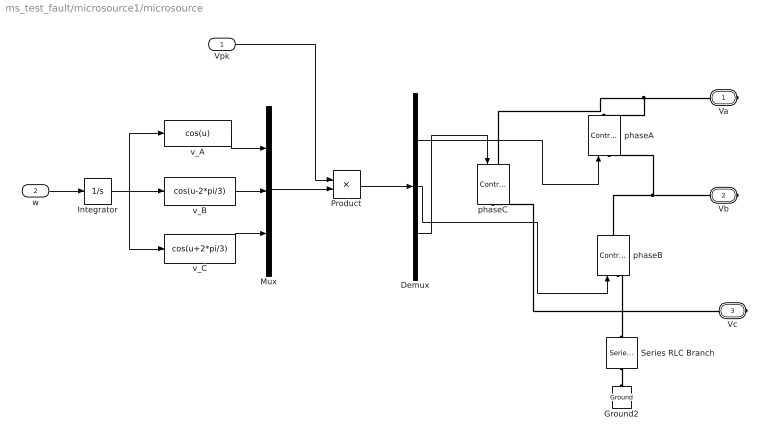
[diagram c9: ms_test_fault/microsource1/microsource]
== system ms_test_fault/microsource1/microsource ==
  Vpk : Inport  OutDataType=fixdt(1, 16)  OutScaling=2^0
  w : Inport  Port=2  OutDataType=fixdt(1, 16)  OutScaling=2^0
  Demux : Demux  Outputs=3
  Ground2 : powerlib/Elements/Ground  DialogController=POWERSYS.PowerSysDialog  PhysicalDomain=powersysdomain  SubClassName=unknown  LeftPortType=p1  RightPortType=p1  LConnTagsString=a
  Integrator : Integrator
  Mux : Mux  Inputs=3
  Product : Product  OutDataType=sfix(16)  OutScaling=2^0
  Series RLC Branch : powerlib/Elements/Series RLC Branch  DialogController=POWERSYS.PowerSysDialog  PhysicalDomain=powersysdomain  SubClassName=unknown  LeftPortType=p1  RightPortType=p1  LConnTagsString=__new0  RConnTagsString=__new0  BranchType=C  Resistance=1  Inductance=1e-3  SetiL0=off  InitialCurrent=0  Capacitance=1e-8  Setx0=off  InitialVoltage=0  Measurements=None
  phaseA : powerlib/Electrical Sources/Controlled Voltage Source  DialogController=POWERSYS.PowerSysDialog  SystemSampleTime=-1  Initialize=on  Source_Type=AC  Amplitude=0  Phase=0  Frequency=0  Measurements=None
  phaseB : powerlib/Electrical Sources/Controlled Voltage Source  DialogController=POWERSYS.PowerSysDialog  SystemSampleTime=-1  Initialize=on  Source_Type=AC  Amplitude=0  Phase=0  Frequency=0  Measurements=None
  phaseC : powerlib/Electrical Sources/Controlled Voltage Source  DialogController=POWERSYS.PowerSysDialog  SystemSampleTime=-1  Initialize=on  Source_Type=AC  Amplitude=0  Phase=0  Frequency=0  Measurements=None
  v_A : Fcn  Expr=cos(u)
  v_B : Fcn  Expr=cos(u-2*pi/3)
  v_C : Fcn  Expr=cos(u+2*pi/3)
  Va : PMIOPort  Tag=PMCPort  Port=1  Side=Right
  Vb : PMIOPort  Tag=PMCPort  Port=2  Side=Right
  Vc : PMIOPort  Tag=PMCPort  Port=3  Side=Right
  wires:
  Product/1 -> Demux/1
  Vpk/1 -> Product/1
  Mux/1 -> Product/2
  w/1 -> Integrator/1
  Integrator/1 -> v_A/1, v_B/1, v_C/1
  v_A/1 -> Mux/1
  v_B/1 -> Mux/2
  v_C/1 -> Mux/3
  Demux/1 -> phaseA/1
  Demux/2 -> phaseB/1
  Demux/3 -> phaseC/1
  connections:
  Vb/RConn1 -- phaseB/RConn1 -- phaseA/LConn1
  Va/RConn1 -- phaseC/LConn1 -- phaseA/RConn1
  Vc/RConn1 -- phaseC/RConn1
  Series RLC Branch/RConn1 -- Ground2/LConn1
  Series RLC Branch/LConn1 -- phaseB/LConn1

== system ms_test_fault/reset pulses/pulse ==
  Step : Step  Time=tstart  SampleTime=0
  Step1 : Step  Time=tstart+dt  After=-1  SampleTime=0
  Sum : Sum  Inputs=|++  OutDataType=fixdt(1, 16)  OutScaling=2^0
  Out1 : Outport
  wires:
  Step/1 -> Sum/2
  Step1/1 -> Sum/1
  Sum/1 -> Out1/1

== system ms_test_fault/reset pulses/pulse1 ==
  Step : Step  Time=tstart  SampleTime=0
  Step1 : Step  Time=tstart+dt  After=-1  SampleTime=0
  Sum : Sum  Inputs=|++  OutDataType=fixdt(1, 16)  OutScaling=2^0
  Out1 : Outport
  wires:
  Step/1 -> Sum/2
  Step1/1 -> Sum/1
  Sum/1 -> Out1/1

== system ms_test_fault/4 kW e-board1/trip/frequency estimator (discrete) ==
  v : Inport
  Constant : Constant  Value=60  OutDataType=fixdt(1, 16)  OutScaling=2^0
  Fcn : Fcn  Expr=sin(2*pi*u[1])
  Filter1 : dsparch4/Biquad Filter  Tag=BlockMethodSubSystem  DialogController=dspdialog.BiquadFilter  DialogControllerArgs=DataTag0  IIRFiltStruct=Direct form II  CoeffSource=Specify via dialog  BiQuadCoeffs=[1 -1.36 1 1 -1.78 0.87;1 1 0 1 -0.85 0]  a0Flag=Warning  IC=0  ICnum=0  ICden=0  denAccumFracLength=30  denProdOutputFracLength=30  secondMemoryFracLength=15  roundingMode=Floor  overflowMode=off  ScaleValues=[0.05;0.23;1]  optimizeScaleValues=on  ScaleValueMode=Specify via input port (g)  scaleValueFracLength=14  FilterSource=Specify via dialog  dfiltObjectName=dfilt.df2tsos([1 0.3 0.4],[1 0.1 0.2])
  Gain : Gain  Gain=1/150  ParameterDataType=fixdt(1, 16)  ParameterScaling=2^0  OutDataType=fixdt(1, 16)  OutScaling=2^0  SampleTime=dt
  Product : Product  OutDataType=fixdt(1, 16)  OutScaling=2^0
  Scope : Scope
  Sum : Sum  Inputs=|++  OutDataType=fixdt(1, 16)  OutScaling=2^0
  modulo discrete integrator : Subsystem  mask{dt=dt}
      mask prompts: dt "sample time"
  w : Outport  OutDataType=fixdt(1, 16)  OutScaling=2^0
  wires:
  Fcn/1 -> Product/2
  Constant/1 -> Sum/2
  modulo discrete integrator/1(Out1) -> Fcn/1
  Sum/1 -> modulo discrete integrator/1(In1), w/1
  Product/1 -> Filter1/1
  Filter1/1 -> Scope/1, Sum/1
  v/1 -> Gain/1
  Gain/1 -> Product/1

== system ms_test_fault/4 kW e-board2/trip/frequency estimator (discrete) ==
  v : Inport
  Constant : Constant  Value=60  OutDataType=fixdt(1, 16)  OutScaling=2^0
  Fcn : Fcn  Expr=sin(2*pi*u[1])
  Filter1 : dsparch4/Biquad Filter  Tag=BlockMethodSubSystem  DialogController=dspdialog.BiquadFilter  DialogControllerArgs=DataTag1  IIRFiltStruct=Direct form II  CoeffSource=Specify via dialog  BiQuadCoeffs=[1 -1.36 1 1 -1.78 0.87;1 1 0 1 -0.85 0]  a0Flag=Warning  IC=0  ICnum=0  ICden=0  denAccumFracLength=30  denProdOutputFracLength=30  secondMemoryFracLength=15  roundingMode=Floor  overflowMode=off  ScaleValues=[0.05;0.23;1]  optimizeScaleValues=on  ScaleValueMode=Specify via input port (g)  scaleValueFracLength=14  FilterSource=Specify via dialog  dfiltObjectName=dfilt.df2tsos([1 0.3 0.4],[1 0.1 0.2])
  Gain : Gain  Gain=1/150  ParameterDataType=fixdt(1, 16)  ParameterScaling=2^0  OutDataType=fixdt(1, 16)  OutScaling=2^0  SampleTime=dt
  Product : Product  OutDataType=fixdt(1, 16)  OutScaling=2^0
  Scope : Scope
  Sum : Sum  Inputs=|++  OutDataType=fixdt(1, 16)  OutScaling=2^0
  modulo discrete integrator : Subsystem  mask{dt=dt}
      mask prompts: dt "sample time"
  w : Outport  OutDataType=fixdt(1, 16)  OutScaling=2^0
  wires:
  Fcn/1 -> Product/2
  Constant/1 -> Sum/2
  modulo discrete integrator/1(Out1) -> Fcn/1
  Sum/1 -> modulo discrete integrator/1(In1), w/1
  Product/1 -> Filter1/1
  Filter1/1 -> Scope/1, Sum/1
  v/1 -> Gain/1
  Gain/1 -> Product/1

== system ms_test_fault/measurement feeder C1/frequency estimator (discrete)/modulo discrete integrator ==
  In1 : Inport
  Abs : Abs
  Constant1 : Constant  OutDataType=sfix(16)  OutScaling=2^0
  Discrete-Time Integrator : DiscreteIntegrator  ExternalReset=rising  InitialConditionSource=external  SampleTime=dt  OutDataType=fixdt(1, 16)  OutScaling=2^0  ShowStatePort=on  ICPrevOutput=DiscIntNeverNeededParam  ICPrevScaledInput=DiscIntNeverNeededParam
  Gain1 : Gain  Gain=1+.0001  ParameterDataType=sfix(16)  ParameterScaling=2^0  OutDataType=sfix(16)  OutScaling=2^0
  IC : InitialCondition  Value=0
  Math Function : Math  Operator=rem  OutDataType=sfix(16)  OutScaling=2^0
  Relational Operator : RelationalOperator
  Out1 : Outport
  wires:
  Relational Operator/1 -> Discrete-Time Integrator/2
  Discrete-Time Integrator/State -> Gain1/1
  Gain1/1 -> Abs/1
  Constant1/1 -> Relational Operator/2, Math Function/2
  Abs/1 -> Relational Operator/1, Math Function/1
  In1/1 -> Discrete-Time Integrator/1
  Discrete-Time Integrator/1 -> Out1/1
  IC/1 -> Discrete-Time Integrator/3
  Math Function/1 -> IC/1

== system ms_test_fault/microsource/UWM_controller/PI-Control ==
  In1 : Inport
  Gain : Gain  Gain=.01  ParameterDataType=sfix(16)  ParameterScaling=2^0  OutDataType=sfix(16)  OutScaling=2^0
  Gain1 : Gain  Gain=5  ParameterDataType=sfix(16)  ParameterScaling=2^0  OutDataType=sfix(16)  OutScaling=2^0
  Gain2 : Gain  Gain=750  ParameterDataType=sfix(16)  ParameterScaling=2^0  OutDataType=sfix(16)  OutScaling=2^0
  Integrator1 : Integrator  LimitOutput=on  UpperSaturationLimit=100  LowerSaturationLimit=-100  ZeroCross=off
  Sum4 : Sum  Inputs=|++  OutDataType=sfix(16)  OutScaling=2^0
  Out1 : Outport
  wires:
  Gain/1 -> Sum4/1
  Integrator1/1 -> Sum4/2
  In1/1 -> Gain1/1, Gain/1
  Gain1/1 -> Integrator1/1
  Sum4/1 -> Gain2/1
  Gain2/1 -> Out1/1
